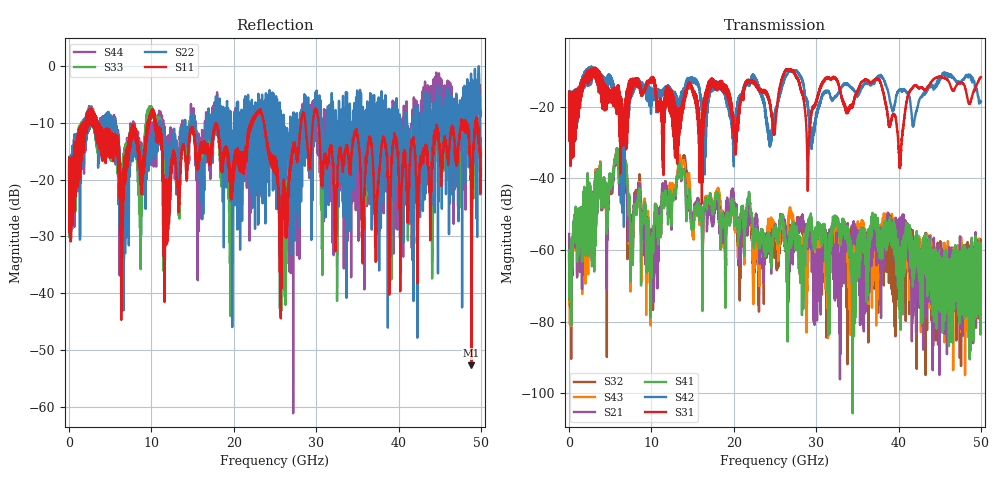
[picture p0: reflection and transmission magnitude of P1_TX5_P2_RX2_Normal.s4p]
!Keysight Technologies,N5225B,MY57041031,A.13.20.10
!Date: Friday, May 31, 2019 11:30:14
!Correction: S11(Full 4 Port(1,2,3,4))
!S12(Full 4 Port(1,2,3,4))
!S13(Full 4 Port(1,2,3,4))
!S14(Full 4 Port(1,2,3,4))
!S21(Full 4 Port(1,2,3,4))
!S22(Full 4 Port(1,2,3,4))
!S23(Full 4 Port(1,2,3,4))
!S24(Full 4 Port(1,2,3,4))
!S31(Full 4 Port(1,2,3,4))
!S32(Full 4 Port(1,2,3,4))
!S33(Full 4 Port(1,2,3,4))
!S34(Full 4 Port(1,2,3,4))
!S41(Full 4 Port(1,2,3,4))
!S42(Full 4 Port(1,2,3,4))
!S43(Full 4 Port(1,2,3,4))
!S44(Full 4 Port(1,2,3,4))
!S4P File: Measurements: <S11,S12,S13,S14>,
!<S21,S22,S23,S24>,
!<S31,S32,S33,S34>,
!<S41,S42,S43,S44>:
# Hz S  dB  R 50.0
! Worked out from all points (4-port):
!   5000 points, 10 MHz to 50 GHz, reference 50 ohm
!   strongest paths, dB at 10 MHz, 12.51 GHz, 25.01 GHz, 37.51 GHz, 50 GHz:
!     S31: -19.4, -23.2, -26.2, -12.3, -11.7
!     S42: -19.4, -16.0, -21.8, -11.4, -18.5
!     S41: -60.1, -46.6, -54.5, -55.0, -58.1
!     S21: -55.5, -46.0, -53.8, -57.5, -62.6
!     S43: -62.0, -42.4, -54.2, -60.1, -72.2
!     S32: -60.3, -43.0, -57.9, -64.9, -72.7
!   lowest |S11| = -52.7 dB at 48.86 GHz (marker M1), VSWR 1.00, Z = 49.8 - j0.0935 ohm
!   |S11| at or under -10 dB: 3.502 GHz to 9.556 GHz (6.054 GHz wide, 92.7 % of centre); 10.5 GHz to 22.11 GHz (11.6 GHz wide, 71.2 % of centre); 30.29 GHz to 47.6 GHz (17.3 GHz wide, 44.4 % of centre)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
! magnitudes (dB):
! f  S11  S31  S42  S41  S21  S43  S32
! 10 MHz  -19.7  -19.4  -19.4  -60.1  -55.5  -62.0  -60.3
! 5.74 GHz  -13.7  -20.4  -16.4  -32.1  -32.3  -32.3  -32.4
! 13.93 GHz  -13.8  -17.6  -18.9  -37.8  -37.5  -35.0  -33.7
! 23.11 GHz  -8.0  -15.7  -14.8  -57.5  -60.7  -64.9  -63.4
! 25.8 GHz  -39.2  -12.6  -15.0  -50.4  -50.9  -50.7  -53.0
! 48.86 GHz  -52.7  -17.7  -11.6  -60.1  -63.9  -62.9  -59.4
! 50 GHz  -18.2  -11.7  -18.5  -58.1  -62.6  -72.2  -72.7
